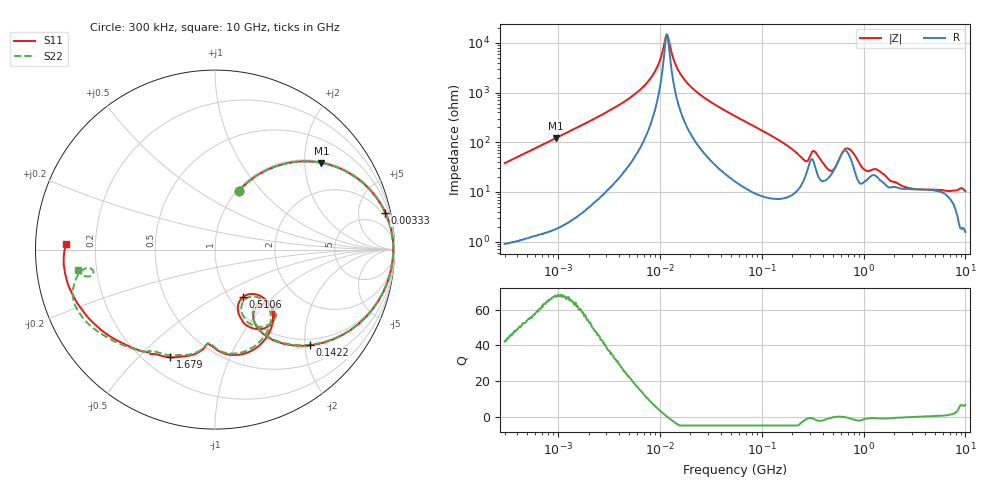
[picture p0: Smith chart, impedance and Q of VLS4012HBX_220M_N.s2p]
! S-Parameter Data Generated by TDK Corporation
! Copyright(C) 2023 TDK Corporation.
! All Rights Reserved.
! TDK P/N: VLS4012HBX-220M-N (Inductor)
! Property: L=22uH at 1MHz
! Size(LxWxT): 4x4x1.2mm
! Model Type: s2p (Touchstone File Format Version 1.0)
! Frequency: DC=Yes Start=0.3MHz Stop=10000MHz 802points Log-sweep
! Model Generated on June 16, 2023
! Port Assignments:
!  1 ---@@@--- 2
! Applicable Conditions:
!  Temperature = 25 degC
!  DC Bias Current = 0 A
!  Small Signal Operation
! Terms and conditions regarding TDK Simulation Models
! (1)This simulation model is being provided solely for informational purposes. Please refer to the specifications of the products in terms of detailed characteristics of such products.
! (2)In no event shall TDK Corporation of any of its subsidiaries be liable for any loss or damage arising, directly or indirectly,
!  From any information contained in this simulation model, including, but not limited to loss or damages arising from any inaccuracies, omissions or errors in connection with such information.
! (3)Any and all copyrights on this simulation model are owned by TDK Corporation.
!  Duplication or redistribution of this simulation model without prior written permission from TDK Corporation is prohibited.
! (4)This simulation model is subject to any modification or change without any prior notice.
! (5)Neither TDK Corporation nor any of its subsidiaries shall make any warranty, express or implied,
!  Including but not limited to the correctness, implied warranties of merchantability and fitness for a particular purpose with respect to this simulation models.
! (6)The use of this simulation model shall be deemed to have consented to the terms and conditions hereof.
# Hz S MA R 50
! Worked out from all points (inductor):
!   801 points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, 300 kHz to 10 GHz, reference 50 ohm
!   read as one part in series: L = 20.1 uH near 318.3 kHz
!   highest Q = 67.9 at 954.6 kHz (marker M1), where L = 20.2 uH
!   self-resonance near 11.75 MHz
!   S11 on the Smith chart (normalised r, x): 300 kHz: 1.02, +0.76; 3.33 MHz: 1.29, +9.18; 142.2 MHz: 0.86, -2.11; 510.6 MHz: 1.16, -0.68; 1.679 GHz: 0.30, -0.62; 10 GHz: 0.09, +0.02
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300000  0.3512 68.0  0.9278 -20.6  0.9282 -20.6  0.3512 68.0
954628  0.765 39.2  0.6327 -50.0  0.6329 -50.0  0.765 39.2
1713600  0.9043 24.2  0.4118 -64.8  0.4119 -64.8  0.9043 24.2
3330145  0.9707 12.2  0.2143 -76.2  0.2144 -76.2  0.9708 12.2
6727812  0.991 4.2  0.07931 -81.6  0.0793 -81.6  0.991 4.2
9671944  0.9933 1.0  0.02711 -75.6  0.02714 -75.6  0.9934 1.0
1.191229e7  0.9932 -0.7  0.006955 13.9  0.006941 13.9  0.9933 -0.7
1.470778e7  0.9922 -2.5  0.03096 73.9  0.03098 73.9  0.9923 -2.4
1.854358e7  0.99 -4.5  0.06301 78.2  0.06303 78.2  0.9901 -4.5
5.477226e7  0.9468 -19.0  0.2794 68.3  0.2795 68.3  0.947 -18.8
1.42154e8  0.7514 -45.2  0.6166 41.6  0.6167 41.6  0.7513 -44.8
2.476102e8  0.4654 -61.6  0.7807 14.5  0.7809 14.5  0.4604 -61.4
3.126428e8  0.4819 -46.5  0.6319 6.6  0.6321 6.6  0.4694 -43.8
3.644326e8  0.4881 -64.1  0.7369 10.0  0.737 10.0  0.489 -61.2
5.105874e8  0.3069 -59.4  0.7545 -11.1  0.7546 -11.0  0.3238 -57.8
6.821612e8  0.5336 -53.8  0.5385 -10.8  0.5386 -10.8  0.5308 -55.6
8.070667e8  0.6023 -74.4  0.6192 -3.7  0.6194 -3.7  0.5913 -74.4
9.560117e8  0.5529 -89.7  0.7151 -12.2  0.7152 -12.2  0.5463 -89.9
1.679152e9  0.6505 -112.7  0.6298 -34.9  0.6299 -34.9  0.6451 -114.7
1.767019e9  0.6607 -115.9  0.626 -37.4  0.6261 -37.4  0.6528 -117.8
4.166115e9  0.8063 -153.2  0.3878 -75.1  0.3879 -75.1  0.8086 -147.7
1e10  0.8319 177.9  0.2227 -111.8  0.2227 -111.8  0.7718 -171.4
